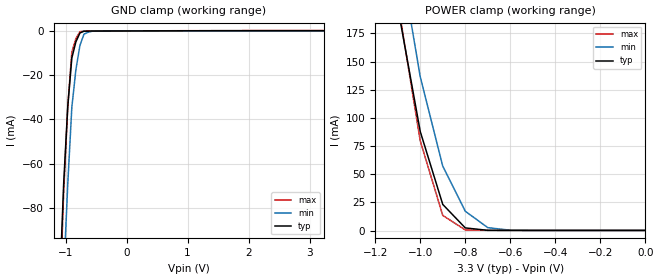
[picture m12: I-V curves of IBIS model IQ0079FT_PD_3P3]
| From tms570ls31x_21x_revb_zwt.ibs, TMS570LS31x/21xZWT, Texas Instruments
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|   Model Cell IQ0079FT_PD_3P3
|IQ0079FT_PD_3P3
[Model]   IQ0079FT_PD_3P3
Model_type   Input
Polarity   Non-Inverting
Vinl =  1.15
Vinh =  1.55
C_comp   1.2p   1.2p   1.2p
[Model Spec]
Vinl   1.15   1.02   1.28
Vinh   1.55   1.45   1.65
[Temperature Range]   25   155   -40
[Voltage Range]   3.3   2.97   3.63
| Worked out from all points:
|   GND clamp passes 1 mA (typ) near -0.77 V on its own axis
|   POWER clamp passes 1 mA (typ) near -0.74 V on its own axis
[POWER_clamp]
|   voltage   I(typ)   I(min)   I(max)
-3.3V     3.541A     4.385A     3.783A
-1.1V     198.8mA    255.1mA    203.5mA
-1.067V   161.8mA    215.6mA    162.2mA
-1.033V   124.9mA    176.1mA    120.9mA
-1V       87.98mA    136.6mA    79.67mA
-900mV    23.19mA    57.17mA    13.42mA
-800mV    2.329mA    17.13mA    516.8uA
-700mV    165.6uA    2.555mA    172.4uA
-600mV    98.49uA    264.7uA    168.8uA
0V        96.5uA     44.2uA     168.6uA
[GND_clamp]
|   voltage   I(typ)   I(min)   I(max)
-3.3V     -2.707A    -2.59A     -3.853A
-1.1V     -116mA     -158.3mA   -124.9mA
-1.033V   -68.85mA   -110.6mA   -72.8mA
-966.7mV  -34.25mA   -69.39mA   -34.34mA
-900mV    -12.25mA   -34.63mA   -9.575mA
-833.3mV  -4.958mA   -17.56mA   -3.496mA
-766.7mV  -914.6uA   -6.492mA   -337.7uA
-700mV    -116.1uA   -1.429mA   -100.1uA
-566.7mV  -52.65uA   -136.8uA   -76.88uA
3.233V    96.49uA    44.32uA    168.5uA
